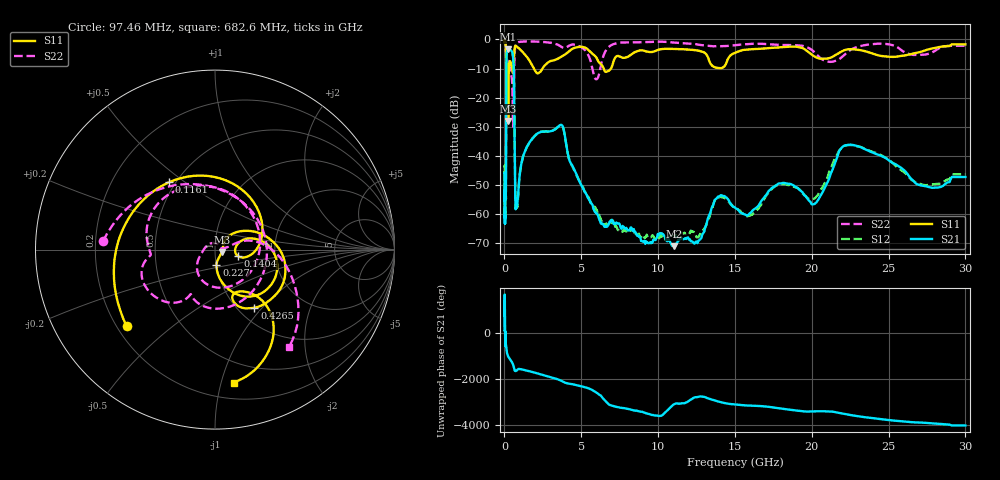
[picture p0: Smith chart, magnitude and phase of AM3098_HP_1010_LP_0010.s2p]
! Date/Time: Thu, Feb 28, 2019 8:41 AM
! Network Analyzer: Agilent Technologies E8364B Rev: A.07.50.67
! Sweep from 0.010 to 30.000 GHz, 1601 Points, Sweep Type: LOG
! Power Supply: 5.022 V, 0.002 A
# Hz S DB R 50
!freq MagS11 AngS11 MagS21 AngS21 MagS12 AngS12 MagS22 AngS22
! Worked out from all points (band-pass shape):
!   1601 points, 10 MHz to 30 GHz, reference 50 ohm
!   highest |S21| = -3.36 dB at 238.7 MHz (marker M1); lowest = -71.1 dB at 11.03 GHz (marker M2)
!   |S21| within 3 dB of the highest: 133 MHz to 566.8 MHz (433.8 MHz wide, 124 % of centre)
!   lowest |S11| = -28.1 dB at 238.7 MHz (marker M3), VSWR 1.08, Z = 53.8 - j1.48 ohm
!   |S11| at or under -10 dB: 199.6 MHz to 292.1 MHz (92.5 MHz wide, 37.6 % of centre); 1.91 GHz to 2.477 GHz (566.7 MHz wide, 25.8 % of centre); 6.463 GHz to 6.933 GHz (470.3 MHz wide, 7.02 % of centre)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
!   |S22| runs from -30.1 to -0.5 dB; largest |S21 - S12| = 0.01
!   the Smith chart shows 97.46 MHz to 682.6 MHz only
!   S11 on the Smith chart (normalised r, x): 97.46 MHz: 0.24, -0.36; 116.1 MHz: 0.46, +0.44; 140.4 MHz: 1.29, -0.10; 227 MHz: 1.00, -0.18; 426.5 MHz: 1.19, -0.91; 682.6 MHz: 0.33, -1.10
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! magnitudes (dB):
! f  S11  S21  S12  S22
! 10 MHz  -0.3  -45.8  -45.4  -0.5
! 38.04 MHz  -0.4  -62.1  -58.7  -0.8
! 97.46 MHz  -3.7  -50.0  -50.8  -4.1
! 116.1 MHz  -6.9  -18.7  -18.7  -10.6
! 140.4 MHz  -17.5  -5.1  -5.1  -11.0
! 144.7 MHz  -19.0  -4.8  -4.7  -10.8
! 186.8 MHz  -8.7  -3.9  -3.9  -7.1
! 227 MHz  -21.1  -3.4  -3.4  -8.8
! 238.7 MHz  -28.1  -3.4  -3.3  -8.9
! 426.5 MHz  -8.2  -3.7  -3.7  -11.9
! 550.5 MHz  -11.5  -5.6  -5.5  -28.5
! 617.6 MHz  -6.2  -13.5  -13.5  -13.7
! 682.6 MHz  -2.5  -46.4  -46.2  -3.3
! 825.6 MHz  -2.5  -57.0  -57.6  -1.2
! 2.084 GHz  -11.5  -32.6  -32.6  -0.7
! 3.723 GHz  -5.9  -29.4  -29.5  -2.6
! 5.989 GHz  -6.3  -59.8  -58.9  -13.7
! 7.926 GHz  -6.2  -64.8  -66.1  -1.0
! 11.03 GHz  -3.3  -71.1  -67.4  -1.1
! 20.2 GHz  -5.9  -56.5  -54.7  -4.6
! 22.67 GHz  -3.4  -36.3  -36.3  -3.2
! 30 GHz  -1.7  -47.3  -46.4  -2.2
